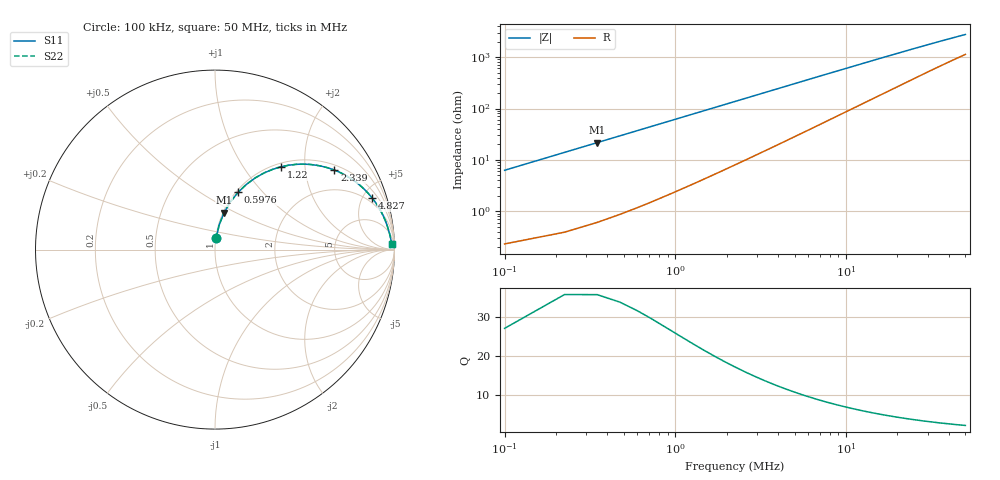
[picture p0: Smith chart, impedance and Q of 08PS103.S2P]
! Coilcraft 0805PS-103 Power Chip Inductor
! 5 February 2003
# MHZ S MA R 50
!Freq  MagS11  AngS11  MagS21  AngS21  MagS12  AngS12  MagS22  AngS22
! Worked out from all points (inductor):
!   403 points, 100 kHz to 50 MHz, reference 50 ohm
!   read as one part in series: L = 9.9 uH near 348.8 kHz
!   highest Q = 29.6 at 348.8 kHz (marker M1), where L = 9.92 uH
!   S11 on the Smith chart (normalised r, x): 100 kHz: 1.00, +0.13; 597.6 kHz: 1.02, +0.74; 1.22 MHz: 1.06, +1.51; 2.339 MHz: 1.17, +2.87; 4.827 MHz: 1.54, +5.87; 50 MHz: 24, +50
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0.1  0.06261 84.3  0.9957 -3.6  0.9957 -3.6  0.06261 84.3
0.2244  0.1384 80.4  0.9865 -8.0  0.9865 -8.0  0.1384 80.4
0.3488  0.2113 76.2  0.9715 -12.2  0.9715 -12.2  0.2113 76.2
0.4732  0.2802 72.0  0.9517 -16.3  0.9517 -16.3  0.2802 72.0
0.5976  0.3445 68.0  0.9279 -20.1  0.9279 -20.1  0.3445 68.0
0.8464  0.4578 60.7  0.8727 -27.2  0.8727 -27.2  0.4578 60.7
1.2196  0.5901 51.4  0.7827 -36.1  0.7827 -36.1  0.5901 51.4
1.7172  0.7093 42.0  0.67 -45.1  0.67 -45.1  0.7093 42.0
2.3392  0.7991 33.7  0.5555 -52.9  0.5555 -52.9  0.7991 33.7
2.8368  0.8434 28.9  0.4842 -57.3  0.4842 -57.3  0.8434 28.9
3.3344  0.8735 25.2  0.4273 -60.6  0.4273 -60.6  0.8735 25.2
3.9564  0.8991 21.7  0.3713 -63.7  0.3713 -63.7  0.8991 21.7
4.8272  0.9219 18.1  0.3127 -66.6  0.3127 -66.6  0.9219 18.1
6.4444  0.9448 13.9  0.2409 -69.9  0.2409 -69.9  0.9448 13.9
8.4348  0.9585 10.7  0.1875 -71.9  0.1875 -71.9  0.9585 10.7
12.1668  0.9699 7.5  0.1325 -73.1  0.1325 -73.1  0.9699 7.5
16.7696  0.9759 5.5  0.09765 -73.0  0.09765 -73.0  0.9759 5.5
20.626  0.9785 4.5  0.08025 -72.2  0.08025 -72.2  0.9785 4.5
25.1044  0.9805 3.7  0.0667 -71.1  0.0667 -71.1  0.9805 3.7
33.4392  0.9826 2.8  0.05116 -68.8  0.05116 -68.8  0.9826 2.8
41.774  0.9839 2.2  0.04185 -66.3  0.04185 -66.3  0.9839 2.2
50  0.9848 1.9  0.03576 -63.9  0.03576 -63.9  0.9848 1.9
